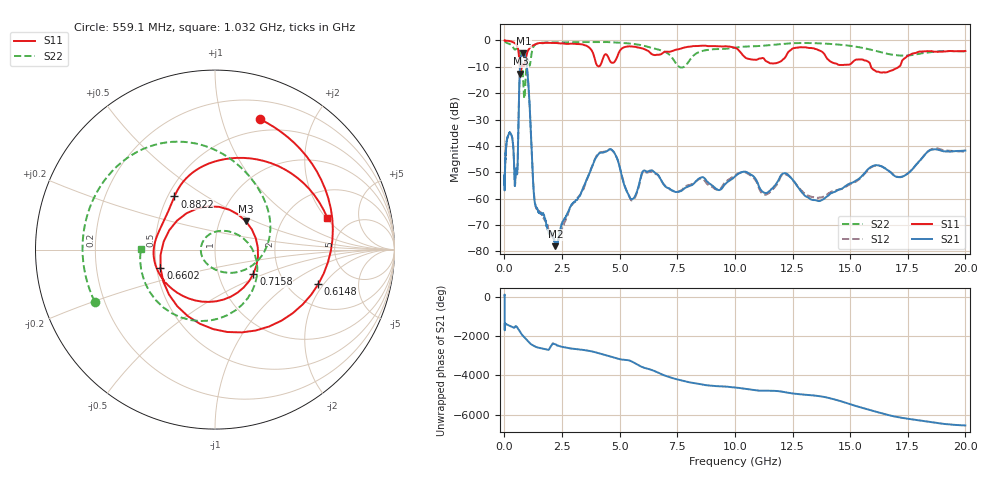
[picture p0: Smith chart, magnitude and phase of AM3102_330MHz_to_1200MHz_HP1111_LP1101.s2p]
! Date/Time: Tue, Sep 11, 2018 5:24 PM
! Network Analyzer: Agilent Technologies E8362B Rev: A.07.50.63
! Sweep from 0.010 to 20.000 GHz, 1601 Points, Sweep Type: LOG
! Power Supply: 4.949 V, 0.001 A
# Hz S DB R 50
!freq MagS11 AngS11 MagS21 AngS21 MagS12 AngS12 MagS22 AngS22
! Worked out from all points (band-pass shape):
!   1601 points, 10 MHz to 20 GHz, reference 50 ohm
!   highest |S21| = -4.92 dB at 825.4 MHz (marker M1); lowest = -78.0 dB at 2.217 GHz (marker M2)
!   |S21| within 3 dB of the highest: 698.8 MHz to 944.8 MHz (246 MHz wide, 29.9 % of centre)
!   lowest |S11| = -12.6 dB at 695.6 MHz (marker M3), VSWR 1.61, Z = 66.7 + j22.1 ohm
!   |S11| at or under -10 dB: 661.1 MHz to 755.6 MHz (94.5 MHz wide, 13.3 % of centre); 15.91 GHz to 17.11 GHz (1.208 GHz wide, 7.32 % of centre)
!   |S22| runs from -22.0 to -0.2 dB; largest |S21 - S12| = 0.0068
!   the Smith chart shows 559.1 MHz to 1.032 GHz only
!   S11 on the Smith chart (normalised r, x): 559.1 MHz: 0.38, +1.34; 614.8 MHz: 2.89, -1.77; 660.2 MHz: 0.52, -0.12; 715.8 MHz: 1.47, -0.42; 882.2 MHz: 0.54, +0.37; 1.032 GHz: 3.39, +2.06
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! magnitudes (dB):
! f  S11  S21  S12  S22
! 10 MHz  0.0  -52.0  -51.0  -0.2
! 35.55 MHz  -0.1  -46.6  -46.7  -0.5
! 126.4 MHz  -0.2  -37.0  -37.1  -1.0
! 331.5 MHz  -0.5  -36.5  -36.5  -2.0
! 447.2 MHz  -1.0  -54.4  -54.3  -3.5
! 559.1 MHz  -2.3  -50.3  -50.2  -2.7
! 614.8 MHz  -4.3  -29.4  -29.5  -2.7
! 660.2 MHz  -9.9  -13.8  -13.9  -3.9
! 695.6 MHz  -12.6  -8.2  -8.2  -5.8
! 715.8 MHz  -11.9  -6.8  -6.8  -6.9
! 825.4 MHz  -9.7  -4.9  -5.0  -16.7
! 882.2 MHz  -8.6  -5.6  -5.7  -21.3
! 1.032 GHz  -3.7  -15.5  -15.5  -7.7
! 1.296 GHz  -1.6  -59.9  -59.5  -2.0
! 1.59 GHz  -1.0  -65.4  -65.6  -0.9
! 2.217 GHz  -0.9  -78.0  -76.8  -0.7
! 4.171 GHz  -9.3  -42.7  -42.4  -0.6
! 5.652 GHz  -2.4  -59.3  -59.7  -1.4
! 6.245 GHz  -4.0  -49.7  -50.0  -2.5
! 7.697 GHz  -2.9  -57.0  -56.7  -10.3
! 13.61 GHz  -3.6  -60.9  -59.8  -1.1
! 20 GHz  -4.0  -41.8  -42.2  -4.2
